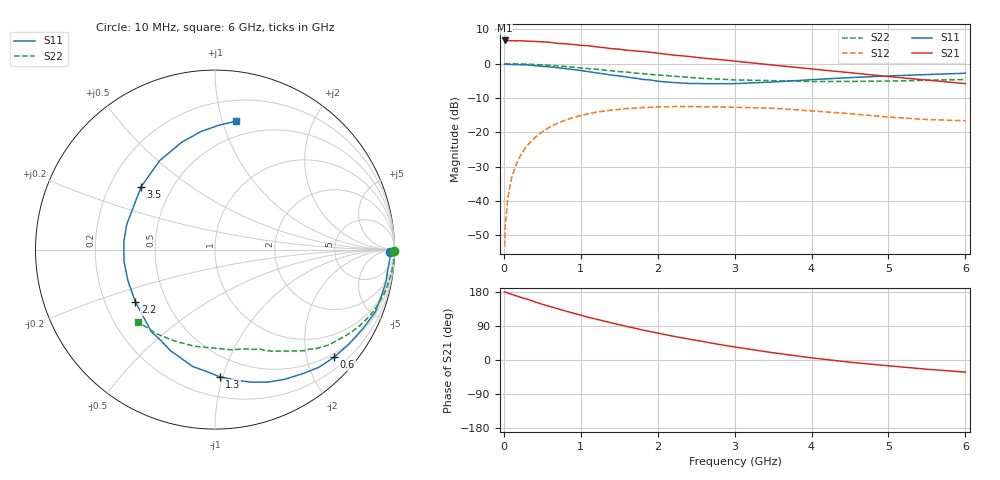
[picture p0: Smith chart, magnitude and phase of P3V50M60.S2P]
! SIEMENS Small Signal Semiconductors
! BFP181
! Si NPN RF Bipolar Junction Transistor in SOT143
! VCE = 0.5 V  IC = 0.6 mA
! Common Emitter S-Parameters:  March  1996
# GHz  S  MA  R  50
!  f  S11  S21  S12  S22
! GHz  MAG  ANG  MAG  ANG  MAG  ANG  MAG  ANG
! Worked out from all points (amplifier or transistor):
!   36 points, 10 MHz to 6 GHz, reference 50 ohm
!   highest |S21| = 6.7 dB at 10 MHz (marker M1)
!   |S21| within 3 dB of that: start of sweep to 1.681 GHz
!   unconditionally stable (mu >= 1): 3.105 GHz to end of sweep
!   at 250 MHz: K = 0.09, MSG = 16.1 dB, |S12| = -25.5 dB
!   at 1.4 GHz: K = 0.52, MSG = 8.9 dB, |S12| = -13.5 dB
!   at 6 GHz: K = 1.67, MAG = 0.6 dB, |S12| = -16.6 dB
!   S11 on the Smith chart (normalised r, x): 10 MHz: 60, -33; 600 MHz: 0.42, -2.54; 1.3 GHz: 0.34, -0.98; 2.2 GHz: 0.33, -0.27; 3.5 GHz: 0.33, +0.33; 6 GHz: 0.37, +1.11
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0.01  0.9747 -0.8  2.174 179.8  0.0022 84.4  0.9982 -0.4
0.02  0.9798 -1.3  2.164 179.4  0.0045 87.8  0.9974 -0.8
0.05  0.9751 -3.2  2.158 176.8  0.0109 88.9  0.9972 -1.9
0.1  0.9689 -7.2  2.157 173.5  0.0214 84.7  0.9991 -3.8
0.15  0.9695 -10.7  2.137 170.2  0.0319 82.1  0.9937 -5.6
0.25  0.9606 -17.9  2.142 163.4  0.0529 77.8  0.9866 -9.4
0.3  0.9586 -21.2  2.126 161.0  0.0636 75.2  0.9829 -11.3
0.4  0.9344 -28.0  2.104 153.7  0.0833 70.0  0.9735 -14.9
0.6  0.8942 -42.1  2.043 141.1  0.12 60.1  0.9441 -22.0
0.8  0.8454 -55.0  1.943 129.4  0.1504 51.3  0.9075 -28.3
1.1  0.7637 -75.2  1.817 112.7  0.1865 39.0  0.8455 -36.9
1.3  0.7089 -87.9  1.709 102.8  0.2038 31.4  0.8068 -42.2
1.5  0.6631 -100.8  1.622 93.1  0.2153 25.0  0.7648 -46.5
1.8  0.5897 -120.7  1.503 79.3  0.2291 17.0  0.7148 -52.1
2.2  0.5312 -146.6  1.334 62.8  0.2369 6.6  0.6573 -59.5
2.4  0.515 -160.2  1.274 55.4  0.2377 1.7  0.6324 -63.0
2.8  0.5097 175.1  1.146 41.0  0.2346 -5.7  0.5959 -69.0
3.5  0.5401 139.7  0.953 19.1  0.2241 -16.9  0.5654 -80.7
4  0.5835 122.0  0.837 5.7  0.205 -23.1  0.5486 -91.0
4.5  0.6257 107.4  0.738 -5.9  0.1869 -28.3  0.5508 -102.3
5.5  0.6929 88.3  0.576 -24.4  0.1537 -28.3  0.5715 -125.1
6  0.7249 80.8  0.512 -32.0  0.1472 -25.5  0.5874 -136.8
